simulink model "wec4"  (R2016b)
settings: Solver=ode4  StartTime=0  StopTime=1000  FixedStep=0.005  MaxStep=0.005  RelTol=1e-3  EnableMultiTasking=on
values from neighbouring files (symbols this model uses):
  arAdaptiveLawData = 1/2*zModelSimple.zModelPto.arFreq.*     zModelSimple.zModelPto.arMagnitude./     cos(zModelSimple.zModelPto.arPhase*pi/180+pi/2)    [IMPACT_Control.m]
  arAdaptiveLawDataX = 1/2*zModelSimpleX.zModelPto.arFreq.*         zModelSimpleX.zModelPto.arMagnitude./         cos(zModelSimpleX.zModelPto.arPhase*pi/180+pi/2)    [IMPACT_Control.m]
  arControllerRampGain = [0,0,1,1]    [IMPACT_Control.m]
  arControllerRampTime = [0 rStartRampTime rStartRampTime+rRampTimeLength 8000]    [IMPACT_Control.m]
  arEkfInitialisation = zeros(1,11)    [IMPACT_Control.m]
  arEkfInitialisationX = zeros(1,11)    [IMPACT_Control.m]
  arFrequency = zModelSimple.zModelPto.arFreq    [IMPACT_Control.m]
  arFrequencyRange = zModelSimple.zModelPto.arFreq    [IMPACT_Control.m]
  arFrequencyX = zModelSimpleX.zModelPto.arFreq    [IMPACT_Control.m]
  arImpedance = 1./zModelSimple.zModelPto.arMagnitude./zModelSimple.zModelPto.arFreq    [IMPACT_Control.m]
  arImpedanceX = 1./zModelSimpleX.zModelPto.arMagnitude./zModelSimpleX.zModelPto.arFreq    [IMPACT_Control.m]
  CentralPTOPreload = -1.6113e+07    (= -16113000)    [wecSimInputFile.m]
  F1 = [4.243 2.375 -12.243]    [wecSimInputFile.m]
  F2 = [4.243 -2.375 -12.243]    [wecSimInputFile.m]
  F3 = [-4.243 -2.375 -12.243]    [wecSimInputFile.m]
  F4 = [-4.243 2.375 -12.243]    [wecSimInputFile.m]
  FC = [0 0 -14]    [wecSimInputFile.m]
  iAdaptiveDamping = 0    [wec4IMPACT_Project.m]    (also in IMPACT_Control.m = handles.iAdaptiveDamping; wec1_IMPACT_Project.m; wec2_IMPACT_Project.m; wec3_IMPACT_Project.m)
  iControlType = 2    [wec4IMPACT_Project.m]    (also in IMPACT_Control.m = handles.iControlType; wec1_IMPACT_Project.m = 1; wec2_IMPACT_Project.m = 1; wec3_IMPACT_Project.m = 1)
  iPtoPositionConstraint = 1    [wec4IMPACT_Project.m]    (also in IMPACT_Control.m = handles.iPtoPositionConstraint; wec1_IMPACT_Project.m = 0; wec2_IMPACT_Project.m; wec3_IMPACT_Project.m)
  iSensorNoise = 0    [IMPACT_Control.m]
  m = m+1    (= 2)    [checkParamFile.m]
  PTOrotation = atan((T1(2)-F1(2))/(T1(1)-F1(1)))    [wecSimInputFile.m]
  rCogFloater = -8    [wec4_IMPACT_Model.m]    (also in paramInitial.m = get( handles.edit_rCogFloater, 'String' ); wec1_IMPACT_Model.m = -18; wec2_IMPACT_Model.m = -8.5; wec3_IMPACT_Model.m = -0.7)
  rCogSpar = -36.6    [wec4_IMPACT_Model.m]    (also in paramInitial.m = get( handles.edit_rCogSpar, 'String' ); wec3_IMPACT_Model.m = -21.3; wec3_IMPACT_Model2.m = -21.3)
  rDisplacementLimit = 10.000000    (= 10)    [wec4IMPACT_Project.m]    (also in IMPACT_Control.m = getValue(handles.edit_displacementLimit); wec1_IMPACT_Project.m; wec2_IMPACT_Project.m; wec3_IMPACT_Project.m = 3)
  rDisplacementLimitX = 10.000000    (= 10)    [wec4IMPACT_Project.m]    (also in IMPACT_Control.m = getValue(handles.edit_displacementLimitX); wec1_IMPACT_Project.m = 0; wec2_IMPACT_Project.m; wec3_IMPACT_Project.m = 0)
  rGainForAntiWIndUp = tfControllerDiscrete.rGain    [IMPACT_Control.m]
  rGainForAntiWIndUpX = tfControllerXDiscrete.rGain    [IMPACT_Control.m]
  rMaxForcePto = 300000000.000000    (= 300000000)    [wec4IMPACT_Project.m]    (also in IMPACT_Control.m = getValue(handles.edit_maxForcePto); wec1_IMPACT_Project.m = 1e+15; wec2_IMPACT_Project.m = 1e+15; wec3_IMPACT_Project.m = 1000000000)
  rMinForcePto = -300000000.000000    (= -300000000)    [wec4IMPACT_Project.m]    (also in IMPACT_Control.m = getValue(handles.edit_minForcePto); wec1_IMPACT_Project.m = -1e+15; wec2_IMPACT_Project.m = -1e+15; wec3_IMPACT_Project.m = -1000000000)
  rMooringX = 20000    [wec4_IMPACT_Model.m]    (also in paramInitial.m = get( handles.edit_rMooringX, 'String' ); wec3_IMPACT_Model.m = 10000; wec3_IMPACT_Model2.m = 10000)
  rMooringZ = 10000    [wec4_IMPACT_Model.m]    (also in paramInitial.m = get( handles.edit_rMooringZ, 'String' ); wec3_IMPACT_Model.m = 0; wec3_IMPACT_Model2.m = 0)
  rOutputSampleTime = 0.010000    (= 0.01)    [wec4IMPACT_Project.m]    (also in IMPACT_Control.m = getValue(handles.edit_outputSampleTime); wec1_IMPACT_Project.m; wec2_IMPACT_Project.m; wec3_IMPACT_Project.m)
  rPassiveDampingGain = -604830.000000    (= -604830)    [wec4IMPACT_Project.m]    (also in IMPACT_Control.m = getValue(handles.edit_gainPLD); wec1_IMPACT_Project.m = -214018.1537; wec2_IMPACT_Project.m = -1948070; wec3_IMPACT_Project.m = -519390)
  rPassiveDampingGainX = -278660.000000    (= -278660)    [wec4IMPACT_Project.m]    (also in IMPACT_Control.m = getValue(handles.edit_gainPLDX); wec1_IMPACT_Project.m = 0; wec2_IMPACT_Project.m = 0; wec3_IMPACT_Project.m = 0)
  rTetherPretension = 1.6113e+07    (= 16113000)    [wec4_IMPACT_Model.m]    (also in paramInitial.m = get( handles.edit_rTetherPretension, 'String' ); wec3_IMPACT_Model.m = 0; wec3_IMPACT_Model2.m = 0)
  rTetherSpring = 500000    [wec4_IMPACT_Model.m]    (also in paramInitial.m = get( handles.edit_rTetherSpring, 'String' ); wec3_IMPACT_Model.m = 0; wec3_IMPACT_Model2.m = 0)
  rUpperFrequencyLimit = EKFFloater.upperFreq    [IMPACT_Control.m]
  rXf = 4.243    [wec4AdditionalParams.m]
  rXs = 16.075    [wec4AdditionalParams.m]
  rYf = 2.375    [wec4AdditionalParams.m]
  rYs = 16.075    [wec4AdditionalParams.m]
  rZf = 4.243    [wec4AdditionalParams.m]
  rZs = 2.4350    (= 2.435)    [wec4AdditionalParams.m]
  rZTetherF = 6    [wec4AdditionalParams.m]
  rZTetherS = 2.4350    (= 2.435)    [wec4AdditionalParams.m]
  s = tf('s')    [wec4_IMPACT_Model.m]    (also in IMPACT_Control.m; wec1_IMPACT_Model.m; wec2_IMPACT_Model.m; wec3_IMPACT_Model.m)
  SidePTO1Preload = PreloadPTOCorner    (= 0)    [wecSimInputFile.m]
  SidePTO2Preload = PreloadPTOCorner    (= 0)    [wecSimInputFile.m]
  SidePTO3Preload = PreloadPTOCorner    (= 0)    [wecSimInputFile.m]
  SidePTO4Preload = PreloadPTOCorner    (= 0)    [wecSimInputFile.m]
  simu = simulationClass()    [wecSimInputFile.m]
  T1 = [16.075 16.075 -34.165]    [wecSimInputFile.m]
  T2 = [16.075 -16.075 -34.165]    [wecSimInputFile.m]
  T3 = [-16.075 -16.075 -34.165]    [wecSimInputFile.m]
  T4 = [-16.075 16.075 -34.165]    [wecSimInputFile.m]
  TC = [0 0 -34.165]    [wecSimInputFile.m]
  waves = waveClass('irregular')    [wecSimInputFile.m]
  Z = magPhaseToComplex(zModelTf)    [IMPACT_Control.m]
undefined symbols (not defined in the file or in its folder): arControllerDiscreteDen, arControllerDiscreteNum, arControllerDiscreteXDen, arControllerDiscreteXNum, arExcForceFloaterDen, arExcForceFloaterNum, arExcForceFloaterXDen, arExcForceFloaterXNum, arExcForceSparDen, arExcForceSparNum, arExcForceSparXDen, arExcForceSparXNum, arFexcFloaterDen, arFexcFloaterNum, arFexcFloaterXDen, arFexcFloaterXNum, arFexcSparDen, arFexcSparNum, arFexcSparXDen, arFexcSparXNum, Body, body, constraint, CTTime, deg, Elements, geometry, IRKB, kg, lenJ, mooring, N, pto, rAccelerationGainFloater, rAccelerationGainFloaterX, rAccelerationGainSpar, rAccelerationGainSparX, rad, rBuoyancyGainFloater, rBuoyancyGainFloaterX, rBuoyancyGainSpar, rBuoyancyGainSparX, rDampingGainFloater, rDampingGainFloaterX, rDampingGainSpar, rDampingGainSparX, Rigid, rMaxFocePto, wec4_float, wec4_reactor, WECSim_Lib, X, Y
libraries: nesl_utility x380, sm_lib x170, vrlib x91, simulink x12, WECSim_Lib x4
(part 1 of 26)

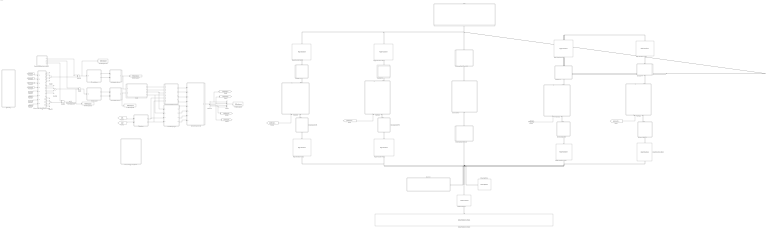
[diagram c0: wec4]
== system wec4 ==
  Central tether : Subsystem
  Demux1 : Demux
  EKFs : Subsystem
  Excitation force : Subsystem
  Excitation force1 : Subsystem
  Float : Subsystem  AncestorBlock=WECSim_Lib/Body Elements/Rigid Body  Variant=on
  Floating (3DOF) : WECSim_Lib/Constraints/Floating (3DOF)  constraint=constraint(1)
  Force of Tether in x,y and z1 : Subsystem
  Force of the four PTOs in x,y and z : Subsystem
  Gimbal F1 : Subsystem  AncestorBlock=WECSim_Lib/Constraints/Rotational
  Gimbal F2 : Subsystem  AncestorBlock=WECSim_Lib/Constraints/Rotational
  Gimbal F3 : Subsystem  AncestorBlock=WECSim_Lib/Constraints/Rotational
  Gimbal F4 : Subsystem  AncestorBlock=WECSim_Lib/Constraints/Rotational
  Global Reference Frame : WECSim_Lib/Frames/Global Reference Frame  waves=waves  simu=simu
  MooringMatrix : WECSim_Lib/Moorings/MooringMatrix  mooring=mooring(1)
  Mux5 : Mux
  OVT : Subsystem
  PTO P1F1 : Subsystem
  PTO P2F2 : Subsystem
  PTO P3F3 : Subsystem
  PTO P4F4 : Subsystem
  Reactor : Subsystem  AncestorBlock=WECSim_Lib/Body Elements/Rigid Body  Variant=on
  Rigid Transform F1P1 : sm_lib/Frames and Transforms/Rigid Transform  TranslationMethod=None  TranslationStandardOffset=0  TranslationLengthUnit=m  TranslationStandardAxis=+Z  TranslationCartesianOffset=[0 0 0]  TranslationROffset=0  TranslationROffsetUnits=m  TranslationZOffset=0  TranslationZOffsetUnits=m  TranslationThetaOffset=0  TranslationThetaOffsetUnits=deg  RotationMethod=StandardAxis  RotationAngleUnits=rad  RotationStandardAxis=+Z  RotationAngle=PTOrotation  RotationArbitraryAxis=[0 0 1]  FollAlignAxisA=+X  BaseAlignAxisA=+Y  FollAlignAxisB=+Y  BaseAlignAxisB=+Z  RotationSequenceAxes=FollowerAxes  RotationSequence=XYX  RotationSequenceAngles=[0 0 0]  RotationSequenceAnglesUnits=deg  RotationMatrix=[1 0 0; 0 1 0; 0 0 1]
  Rigid Transform F2P2 : sm_lib/Frames and Transforms/Rigid Transform  TranslationMethod=None  TranslationStandardOffset=0  TranslationLengthUnit=m  TranslationStandardAxis=+Z  TranslationCartesianOffset=[0 0 0]  TranslationROffset=0  TranslationROffsetUnits=m  TranslationZOffset=0  TranslationZOffsetUnits=m  TranslationThetaOffset=0  TranslationThetaOffsetUnits=deg  RotationMethod=StandardAxis  RotationAngleUnits=rad  RotationStandardAxis=+Z  RotationAngle=-PTOrotation  RotationArbitraryAxis=[0 0 1]  FollAlignAxisA=+X  BaseAlignAxisA=+Y  FollAlignAxisB=+Y  BaseAlignAxisB=+Z  RotationSequenceAxes=FollowerAxes  RotationSequence=XYX  RotationSequenceAngles=[0 0 0]  RotationSequenceAnglesUnits=deg  RotationMatrix=[1 0 0; 0 1 0; 0 0 1]
  Rigid Transform F3P3 : sm_lib/Frames and Transforms/Rigid Transform  TranslationMethod=None  TranslationStandardOffset=0  TranslationLengthUnit=m  TranslationStandardAxis=+Z  TranslationCartesianOffset=[0 0 0]  TranslationROffset=0  TranslationROffsetUnits=m  TranslationZOffset=0  TranslationZOffsetUnits=m  TranslationThetaOffset=0  TranslationThetaOffsetUnits=deg  RotationMethod=StandardAxis  RotationAngleUnits=rad  RotationStandardAxis=+Z  RotationAngle=-pi+PTOrotation  RotationArbitraryAxis=[0 0 1]  FollAlignAxisA=+X  BaseAlignAxisA=+Y  FollAlignAxisB=+Y  BaseAlignAxisB=+Z  RotationSequenceAxes=FollowerAxes  RotationSequence=XYX  RotationSequenceAngles=[0 0 0]  RotationSequenceAnglesUnits=deg  RotationMatrix=[1 0 0; 0 1 0; 0 0 1]
  Rigid Transform F4P4 : sm_lib/Frames and Transforms/Rigid Transform  TranslationMethod=None  TranslationStandardOffset=0  TranslationLengthUnit=m  TranslationStandardAxis=+Z  TranslationCartesianOffset=[0 0 0]  TranslationROffset=0  TranslationROffsetUnits=m  TranslationZOffset=0  TranslationZOffsetUnits=m  TranslationThetaOffset=0  TranslationThetaOffsetUnits=deg  RotationMethod=StandardAxis  RotationAngleUnits=rad  RotationStandardAxis=+Z  RotationAngle=pi-PTOrotation  RotationArbitraryAxis=[0 0 1]  FollAlignAxisA=+X  BaseAlignAxisA=+Y  FollAlignAxisB=+Y  BaseAlignAxisB=+Z  RotationSequenceAxes=FollowerAxes  RotationSequence=XYX  RotationSequenceAngles=[0 0 0]  RotationSequenceAnglesUnits=deg  RotationMatrix=[1 0 0; 0 1 0; 0 0 1]
  Rigid Transform P1F1 : sm_lib/Frames and Transforms/Rigid Transform  TranslationMethod=None  TranslationStandardOffset=0  TranslationLengthUnit=m  TranslationStandardAxis=+Z  TranslationCartesianOffset=[0 0 0]  TranslationROffset=0  TranslationROffsetUnits=m  TranslationZOffset=0  TranslationZOffsetUnits=m  TranslationThetaOffset=0  TranslationThetaOffsetUnits=deg  RotationMethod=StandardAxis  RotationAngleUnits=rad  RotationStandardAxis=+Z  RotationAngle=PTOrotation  RotationArbitraryAxis=[0 0 1]  FollAlignAxisA=+X  BaseAlignAxisA=+Y  FollAlignAxisB=+Y  BaseAlignAxisB=+Z  RotationSequenceAxes=FollowerAxes  RotationSequence=XYX  RotationSequenceAngles=[0 0 0]  RotationSequenceAnglesUnits=deg  RotationMatrix=[1 0 0; 0 1 0; 0 0 1]
  Rigid Transform P2F2 : sm_lib/Frames and Transforms/Rigid Transform  TranslationMethod=None  TranslationStandardOffset=0  TranslationLengthUnit=m  TranslationStandardAxis=+Z  TranslationCartesianOffset=[0 0 0]  TranslationROffset=0  TranslationROffsetUnits=m  TranslationZOffset=0  TranslationZOffsetUnits=m  TranslationThetaOffset=0  TranslationThetaOffsetUnits=deg  RotationMethod=StandardAxis  RotationAngleUnits=rad  RotationStandardAxis=+Z  RotationAngle=-PTOrotation  RotationArbitraryAxis=[0 0 1]  FollAlignAxisA=+X  BaseAlignAxisA=+Y  FollAlignAxisB=+Y  BaseAlignAxisB=+Z  RotationSequenceAxes=FollowerAxes  RotationSequence=XYX  RotationSequenceAngles=[0 0 0]  RotationSequenceAnglesUnits=deg  RotationMatrix=[1 0 0; 0 1 0; 0 0 1]
  Rigid Transform P3F3 : sm_lib/Frames and Transforms/Rigid Transform  TranslationMethod=None  TranslationStandardOffset=0  TranslationLengthUnit=m  TranslationStandardAxis=+Z  TranslationCartesianOffset=[0 0 0]  TranslationROffset=0  TranslationROffsetUnits=m  TranslationZOffset=0  TranslationZOffsetUnits=m  TranslationThetaOffset=0  TranslationThetaOffsetUnits=deg  RotationMethod=StandardAxis  RotationAngleUnits=rad  RotationStandardAxis=+Z  RotationAngle=-pi+PTOrotation  RotationArbitraryAxis=[0 0 1]  FollAlignAxisA=+X  BaseAlignAxisA=+Y  FollAlignAxisB=+Y  BaseAlignAxisB=+Z  RotationSequenceAxes=FollowerAxes  RotationSequence=XYX  RotationSequenceAngles=[0 0 0]  RotationSequenceAnglesUnits=deg  RotationMatrix=[1 0 0; 0 1 0; 0 0 1]
  Rigid Transform P4F4 : sm_lib/Frames and Transforms/Rigid Transform  TranslationMethod=None  TranslationStandardOffset=0  TranslationLengthUnit=m  TranslationStandardAxis=+Z  TranslationCartesianOffset=[0 0 0]  TranslationROffset=0  TranslationROffsetUnits=m  TranslationZOffset=0  TranslationZOffsetUnits=m  TranslationThetaOffset=0  TranslationThetaOffsetUnits=deg  RotationMethod=StandardAxis  RotationAngleUnits=rad  RotationStandardAxis=+Z  RotationAngle=pi-PTOrotation  RotationArbitraryAxis=[0 0 1]  FollAlignAxisA=+X  BaseAlignAxisA=+Y  FollAlignAxisB=+Y  BaseAlignAxisB=+Z  RotationSequenceAxes=FollowerAxes  RotationSequence=XYX  RotationSequenceAngles=[0 0 0]  RotationSequenceAnglesUnits=deg  RotationMatrix=[1 0 0; 0 1 0; 0 0 1]
  Subsystem : Subsystem
  Sum10 : Sum
  Sum12 : Sum  Inputs=+--+
  Sum13 : Sum
  Sum16 : Sum  Inputs=--++
  Sum2 : Sum
  Sum9 : Sum  Inputs=++++
  Terminator3 Rise of the machines : Terminator
  To Workspace10 : ToWorkspace  VariableName=arForceVerticalFloater  SampleTime=rOutputSampleTime
  To Workspace21 : ToWorkspace  VariableName=arTotalPtoForceX  SampleTime=rOutputSampleTime
  To Workspace5 : ToWorkspace  VariableName=arPtoForceDemand  SampleTime=rOutputSampleTime
  To Workspace7 : ToWorkspace  VariableName=arCombinedForceZ  SampleTime=rOutputSampleTime
  To Workspace8 : ToWorkspace  VariableName=arCominedForceX  SampleTime=rOutputSampleTime
  Universal Joint Central : Subsystem  AncestorBlock=WECSim_Lib/Constraints/Rotational
  Universal Joint Central1 : Subsystem  AncestorBlock=WECSim_Lib/Constraints/Rotational
  Universal Joint P1 : Subsystem  AncestorBlock=WECSim_Lib/Constraints/Rotational
  Universal Joint P2 : Subsystem  AncestorBlock=WECSim_Lib/Constraints/Rotational
  Universal Joint P3 : Subsystem  AncestorBlock=WECSim_Lib/Constraints/Rotational
  Universal Joint P4 : Subsystem  AncestorBlock=WECSim_Lib/Constraints/Rotational
  X Excitation : Subsystem
  Z excitation : Subsystem
  controllerSwitching : Subsystem
  "force, energy, and power" : Subsystem
  geometry : Subsystem
  linearDamping1 : Subsystem
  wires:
  [ptoForceDemand1] -> PTO P1F1/1(P1F1_force)
  [ptoForceDemand2] -> PTO P2F2/1(P2F2_force)
  [ptoForceDemand3] -> PTO P3F3/1(P3F3_force)
  [ptoForceDemand4] -> PTO P4F4/1(P4F4_force)
  Force of the four PTOs in x,y and z/7(Fx3) -> Sum16/3
  Force of the four PTOs in x,y and z/8(Fx4) -> Sum16/4
  Force of the four PTOs in x,y and z/6(Fx2) -> Sum16/2
  Force of the four PTOs in x,y and z/1(Fz1) -> Sum9/1
  Force of the four PTOs in x,y and z/3(Fz3) -> Sum9/3
  Force of the four PTOs in x,y and z/4(Fz4) -> Sum9/4
  Force of the four PTOs in x,y and z/2(Fz2) -> Sum9/2
  Force of the four PTOs in x,y and z/10(Fy2) -> Sum12/2
  Force of the four PTOs in x,y and z/12(Fy4) -> Sum12/4
  Force of the four PTOs in x,y and z/9(Fy1) -> Sum12/1
  Force of the four PTOs in x,y and z/11(Fy3) -> Sum12/3
  Sum9/1 -> Sum10/2
  Force of the four PTOs in x,y and z/5(Fx1) -> Sum16/1
  Sum12/1 -> Sum13/2
  Force of Tether in x,y and z1/2(FRx) -> Sum2/1
  Force of Tether in x,y and z1/3(FRy) -> Sum13/1
  Force of Tether in x,y and z1/1(FRz) -> Sum10/1
  Sum10/1 -> Z excitation/1(PTO force Z), To Workspace10/1
  Sum16/1 -> To Workspace21/1, Sum2/2
  Sum2/1 -> X Excitation/1(PTO force X)
  Sum13/1 -> Terminator3 Rise of the machines/1
  EKFs/2(referenceVelocityZ) -> OVT/2(vref_z)
  Mux5/1 -> To Workspace5/1
  EKFs/3(ekfFreqZ) -> linearDamping1/1(ekfFrequencyZ), OVT/3(ekfFreqZ)
  EKFs/1(referenceVelocityX) -> OVT/1(vref_x)
  Demux1/4 -> [ptoForceDemand4], Mux5/4
  Demux1/3 -> [ptoForceDemand3], Mux5/3
  Demux1/2 -> [ptoForceDemand2], Mux5/2
  Demux1/1 -> [ptoForceDemand1], Mux5/1
  Excitation force/1(Combined Fexc) -> EKFs/1(excitationForceZ), To Workspace7/1
  Z excitation/1(floaterExcitation) -> Excitation force/1(Fexc floater)
  Z excitation/2(SparExcitation) -> Excitation force/2(Fexc spar)
  Excitation force1/1(Combined Fexc X) -> To Workspace8/1, EKFs/2(excitationForceX)
  X Excitation/1(floaterExcitation) -> Excitation force1/1(Fexc floater)
  X Excitation/2(SparExcitation) -> Excitation force1/2(Fexc spar)
  [gamma1] -> Force of the four PTOs in x,y and z/1(gamma1)
  [gamma3] -> Force of the four PTOs in x,y and z/3(gamma3)
  [kappa1] -> Force of the four PTOs in x,y and z/5(alpha1)
  [kappa3] -> Force of the four PTOs in x,y and z/7(alpha3)
  [gamma4] -> Force of the four PTOs in x,y and z/4(gamma4)
  [gamma2] -> Force of the four PTOs in x,y and z/2(gamma2)
  [kappa2] -> Force of the four PTOs in x,y and z/6(alpha2)
  [kappa4] -> Force of the four PTOs in x,y and z/8(alpha4)
  controllerSwitching/1(forceDemand) -> Demux1/1
  EKFs/4(ekfFreqX) -> linearDamping1/2(ekfFrequencyX), OVT/4(ekfFreqX)
  OVT/4(forceDemand4) -> controllerSwitching/4(ovtForceDemand4)
  OVT/3(forceDemand3) -> controllerSwitching/3(ovtForceDemand3)
  OVT/2(forceDemand2) -> controllerSwitching/2(ovtForceDemand2)
  OVT/1(forceDemand1) -> controllerSwitching/1(ovtForceDemand1)
  linearDamping1/1(forceDemand1) -> controllerSwitching/5(linearDampingForce1)
  linearDamping1/2(forceDemand2) -> controllerSwitching/6(linearDampingForce2)
  linearDamping1/3(forceDemand3) -> controllerSwitching/7(linearDampingForce3)
  linearDamping1/4(forceDemand4) -> controllerSwitching/8(linearDampingForce4)
  [vel1] -> Subsystem/1(Vel floater 6x1)
  [vel2] -> Subsystem/2(Vel Spar 6x1)
  Subsystem/1("Rel. vel. X ") -> OVT/5(Rel. vel X), linearDamping1/3(Rel. vel X)
  Subsystem/2(Rel. vel. Z) -> OVT/6(Rel. vel. Z), linearDamping1/4(Rel. vel. Z)
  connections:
  Rigid Transform P2F2/LConn1 -- Rigid Transform P1F1/LConn1 -- Rigid Transform P4F4/LConn1 -- Rigid Transform P3F3/LConn1 -- Floating (3DOF)/RConn1 -- Reactor/RConn1 -- MooringMatrix/LConn1 -- Universal Joint Central/LConn1
  Float/RConn1 -- Universal Joint Central1/RConn1 -- Rigid Transform F4P4/LConn1 -- Rigid Transform F3P3/LConn1 -- Rigid Transform F2P2/LConn1 -- Rigid Transform F1P1/LConn1
  PTO P3F3/LConn1 -- Universal Joint P3/RConn1
  Universal Joint P1/LConn1 -- Rigid Transform P1F1/RConn1
  Rigid Transform F1P1/RConn1 -- Gimbal F1/RConn1
  Gimbal F1/LConn1 -- PTO P1F1/RConn1
  PTO P1F1/LConn1 -- Universal Joint P1/RConn1
  Rigid Transform F2P2/RConn1 -- Gimbal F2/RConn1
  Universal Joint P2/LConn1 -- Rigid Transform P2F2/RConn1
  Rigid Transform F3P3/RConn1 -- Gimbal F3/RConn1
  Rigid Transform F4P4/RConn1 -- Gimbal F4/RConn1
  Universal Joint P4/LConn1 -- Rigid Transform P4F4/RConn1
  Gimbal F2/LConn1 -- PTO P2F2/RConn1
  PTO P2F2/LConn1 -- Universal Joint P2/RConn1
  Universal Joint Central1/LConn1 -- Central tether/RConn1
  Central tether/LConn1 -- Universal Joint Central/RConn1
  Gimbal F3/LConn1 -- PTO P3F3/RConn1
  Gimbal F4/LConn1 -- PTO P4F4/RConn1
  Rigid Transform P3F3/RConn1 -- Universal Joint P3/LConn1
  PTO P4F4/LConn1 -- Universal Joint P4/RConn1
  Global Reference Frame/RConn1 -- Floating (3DOF)/LConn1

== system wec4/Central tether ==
  CentralTether_preload : Constant  Value=CentralPTOPreload
  PTO Central visu : Subsystem  AncestorBlock=WECSim_Lib/Body Elements/Rigid Body  Variant=on
  Terminator PTO Central : Terminator
  Translational PTO Actuation Force Central : WECSim_Lib/PTOs/Translational PTO Actuation Force  pto=pto(5)
  Conn1 : PMIOPort  Port=1  Side=Right
  Conn2 : PMIOPort  Port=2  Side=Left
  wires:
  CentralTether_preload/1 -> Translational PTO Actuation Force Central/1
  Translational PTO Actuation Force Central/1 -> Terminator PTO Central/1
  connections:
  Translational PTO Actuation Force Central/RConn1 -- PTO Central visu/RConn1 -- Conn1/RConn1
  Translational PTO Actuation Force Central/LConn1 -- Conn2/RConn1

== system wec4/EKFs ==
  excitationForceZ : Inport
  excitationForceX : Inport  Port=2
  Abs1 : Abs
  Abs2 : Abs
  Clock1 : Clock
  Clock3 : Clock
  Constant1 : Constant  Value=arEkfInitialisation
  Constant2 : Constant  Value=arEkfInitialisationX
  Divide1 : Product  Inputs=**
  Divide4 : Product  Inputs=**
  EKF : MATLAB Function  TreatAsAtomicUnit=on
  EKF1 : MATLAB Function  TreatAsAtomicUnit=on
  Ramp gain : Lookup_n-D  NumberOfTableDimensions=1  BreakpointsForDimension1=[0 5 10 8000]  Table=[0 0 1 1]  InternalRulePriority=Speed  RndMeth=Simplest
  Ramp gain1 : Lookup_n-D  NumberOfTableDimensions=1  BreakpointsForDimension1=[0 5 10 8000]  Table=[0 0 1 1]  InternalRulePriority=Speed  RndMeth=Simplest
  Rate Transition1 : RateTransition  OutPortSampleTimeMultiple=0.01  OutPortSampleTime=rControllerSampleTime
  Rate Transition2 : RateTransition  OutPortSampleTimeMultiple=0.01  OutPortSampleTime=rControllerSampleTime
  Saturation1 : Saturate  UpperLimit=rUpperFrequencyLimit  LowerLimit=0  LinearizeAsGain=off
  Saturation2 : Saturate  UpperLimit=rUpperFrequencyLimit  LowerLimit=0  LinearizeAsGain=off
  Terminator3 : Terminator
  Terminator4 : Terminator
  To Workspace1 : ToWorkspace  VariableName=arPhi0Z  SampleTime=rOutputSampleTime
  To Workspace4 : ToWorkspace  VariableName=arEstimatedExcitationForceZ  SampleTime=rOutputSampleTime
  To Workspace5 : ToWorkspace  VariableName=arEkfAmplitudeZ  SampleTime=rOutputSampleTime
  To Workspace6 : ToWorkspace  VariableName=arEkfFrequencyZ  SampleTime=rOutputSampleTime
  To Workspace7 : ToWorkspace  VariableName=arEstimatedExcitationForceX  SampleTime=rOutputSampleTime
  To Workspace8 : ToWorkspace  VariableName=arEkfAmplitudeX  SampleTime=rOutputSampleTime
  To Workspace9 : ToWorkspace  VariableName=arEkfFrequencyX  SampleTime=rOutputSampleTime
  Transfer Fcn{1..2,4..7,9..10} (8 alike) : TransferFcn  Numerator=[400]  Denominator=[1 40 400]
  V ref X : Subsystem
  "V ref Z " : Subsystem
  referenceVelocityX : Outport
  referenceVelocityZ : Outport  Port=2
  ekfFreqZ : Outport  Port=3
  ekfFreqX : Outport  Port=4
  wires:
  Clock1/1 -> Ramp gain1/1
  Ramp gain1/1 -> Divide1/1
  excitationForceX/1 -> Divide1/2
  Clock3/1 -> Ramp gain/1
  Transfer Fcn5/1 -> To Workspace5/1, "V ref Z "/3(ekfAmplitude)
  EKF/3(rFrequencyOutput) -> Transfer Fcn2/1
  Saturation1/1 -> "V ref Z "/2(ekfFrequency), ekfFreqZ/1, To Workspace6/1
  Constant1/1 -> EKF/2(arEkfInitialisation)
  "V ref Z "/1(referenceVelocity) -> referenceVelocityZ/1
  Abs1/1 -> Saturation1/1
  Transfer Fcn2/1 -> Abs1/1
  excitationForceZ/1 -> Divide4/2
  EKF/1(rPhi0Output) -> To Workspace1/1, Transfer Fcn4/1
  Divide4/1 -> Rate Transition1/1, To Workspace4/1
  Ramp gain/1 -> Divide4/1
  EKF/2(rPhi0StarOutput) -> Transfer Fcn1/1
  Transfer Fcn4/1 -> "V ref Z "/1(phiOut)
  Rate Transition1/1 -> EKF/1(rEstimatedExcitationForce)
  V ref X/1(referenceVelocity) -> referenceVelocityX/1
  EKF/4(rAmplitudeOutput) -> Transfer Fcn5/1
  EKF1/3(rFrequencyOutput) -> Transfer Fcn7/1
  Transfer Fcn10/1 -> V ref X/3(ekfAmplitude), To Workspace8/1
  Transfer Fcn9/1 -> V ref X/1(phiOut)
  Abs2/1 -> Saturation2/1
  Constant2/1 -> EKF1/2(arEkfInitialisation)
  Transfer Fcn6/1 -> Terminator4/1
  EKF1/4(rAmplitudeOutput) -> Transfer Fcn10/1
  EKF1/1(rPhi0Output) -> Transfer Fcn9/1
  Transfer Fcn7/1 -> Abs2/1
  Divide1/1 -> Rate Transition2/1, To Workspace7/1
  EKF1/2(rPhi0StarOutput) -> Transfer Fcn6/1
  Rate Transition2/1 -> EKF1/1(rEstimatedExcitationForce)
  Transfer Fcn1/1 -> Terminator3/1
  Saturation2/1 -> To Workspace9/1, ekfFreqX/1, V ref X/2(ekfFrequency)

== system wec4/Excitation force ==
  Fexc floater : Inport
  Fexc spar : Inport  Port=2
  Add : Sum
  Clock3 : Clock
  Divide1 : Product  Inputs=**
  Divide4 : Product  Inputs=**
  Fexc Floater : TransferFcn  Numerator=arFexcFloaterNum  Denominator=arFexcFloaterDen
  Fexc Spar : TransferFcn  Numerator=arFexcSparNum  Denominator=arFexcSparDen
  Ramp gain : Lookup_n-D  NumberOfTableDimensions=1  BreakpointsForDimension1=[0 5 10 8000]  Table=[0 0 1 1]  InternalRulePriority=Speed  RndMeth=Simplest
  Ramp gain1 : Lookup_n-D  NumberOfTableDimensions=1  BreakpointsForDimension1=[0 20 25 8000]  Table=[0 0 1 1]  InternalRulePriority=Speed  RndMeth=Simplest
  Combined Fexc : Outport
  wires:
  Fexc floater/1 -> Divide4/2
  Fexc Floater/1 -> Add/1
  Fexc Spar/1 -> Add/2
  Add/1 -> Combined Fexc/1
  Clock3/1 -> Ramp gain1/1, Ramp gain/1
  Ramp gain/1 -> Divide4/1
  Divide4/1 -> Fexc Floater/1
  Ramp gain1/1 -> Divide1/2
  Divide1/1 -> Fexc Spar/1
  Fexc spar/1 -> Divide1/1

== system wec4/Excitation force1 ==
  Fexc floater : Inport
  Fexc spar : Inport  Port=2
  Add : Sum
  Clock3 : Clock
  Divide1 : Product  Inputs=**
  Divide4 : Product  Inputs=**
  Fexc Floater X : TransferFcn  Numerator=arFexcFloaterXNum  Denominator=arFexcFloaterXDen
  Fexc Spar X : TransferFcn  Numerator=arFexcSparXNum  Denominator=arFexcSparXDen
  Ramp gain : Lookup_n-D  NumberOfTableDimensions=1  BreakpointsForDimension1=[0 5 10 8000]  Table=[0 0 1 1]  InternalRulePriority=Speed  RndMeth=Simplest
  Ramp gain1 : Lookup_n-D  NumberOfTableDimensions=1  BreakpointsForDimension1=[0 20 25 8000]  Table=[0 0 1 1]  InternalRulePriority=Speed  RndMeth=Simplest
  Combined Fexc X : Outport
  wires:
  Divide1/1 -> Fexc Spar X/1
  Ramp gain1/1 -> Divide1/2
  Divide4/1 -> Fexc Floater X/1
  Ramp gain/1 -> Divide4/1
  Clock3/1 -> Ramp gain1/1, Ramp gain/1
  Add/1 -> Combined Fexc X/1
  Fexc Spar X/1 -> Add/2
  Fexc Floater X/1 -> Add/1
  Fexc floater/1 -> Divide4/2
  Fexc spar/1 -> Divide1/1

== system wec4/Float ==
  note: 1) Add Subsystem or Model blocks as valid variant choices. 2) You cannot connect blocks at this level. At simulation, connectivity is automatically determined, based on the active variant and port name matching.
  Hydrodynamic Body : Subsystem  VariantControl=sv_b1_hydroBody
  Non-Hydro Body : Subsystem  VariantControl=sv_b1_nonHydroBody
  Conn : PMIOPort  Port=1  Side=Right

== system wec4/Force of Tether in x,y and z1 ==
  Constant3 : Constant  Value=-rTetherPretension
  Dzs/2 (2) : Constant  Value=TC(3)
  Dzs/2 (2)1 : Constant  Value=FC(3)
  Gain : Gain  Gain=-rTetherSpring
  Gain1 : Gain  Gain=180/pi
  Math Function{,1..5} (6 alike) : Math  Operator=square
  Mux1 : Mux  Inputs=2
  Mux3 : Mux  Inputs=2
  Mux4 : Mux  Inputs=2
  Product{,1..3} (4 alike) : Product
  Scope{1..4,6,11..12} (7 alike) : Scope
  Selector11 : Selector  InputPortWidth=6  IndexOptions=Index vector (dialog)  Indices=1  OutputSizes=1
  Selector12 : Selector  InputPortWidth=6  IndexOptions=Index vector (dialog)  Indices=2  OutputSizes=1
  Selector13 : Selector  InputPortWidth=6  IndexOptions=Index vector (dialog)  Indices=3  OutputSizes=1
  Selector14 : Selector  InputPortWidth=6  IndexOptions=Index vector (dialog)  Indices=1  OutputSizes=1
  Selector15 : Selector  InputPortWidth=6  IndexOptions=Index vector (dialog)  Indices=2  OutputSizes=1
  Selector16 : Selector  InputPortWidth=6  IndexOptions=Index vector (dialog)  Indices=3  OutputSizes=1
  Sqrt : Sqrt
  Sqrt1 : Sqrt
  Subsystem2 : Subsystem
  Sum10 : Sum
  Sum11 : Sum  Inputs=-+
  Sum2 : Sum  Inputs=-+
  Sum31 : Sum  Inputs=+++
  Sum{4,6..8} (4 alike) : Sum  Inputs=+-
  Sum9 : Sum  Inputs=+++
  Trigonometric Function : Trigonometry  Operator=atan2
  Trigonometric Function1 : Trigonometry  Operator=atan2
  Trigonometric Function2 : Trigonometry  Operator=cos
  Trigonometric Function3 : Trigonometry  Operator=cos
  Trigonometric Function4 : Trigonometry
  Trigonometric Function5 : Trigonometry
  FRz : Outport
  FRx : Outport  Port=2
  FRy : Outport  Port=3
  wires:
  Trigonometric Function1/1 -> Trigonometric Function5/1, Mux1/2, Trigonometric Function3/1
  Trigonometric Function/1 -> Mux1/1, Trigonometric Function4/1, Trigonometric Function2/1
  Trigonometric Function2/1 -> Product/1
  Trigonometric Function3/1 -> Product/2
  Product/1 -> Product2/2  "Proportion of force in Z direction"
  Trigonometric Function4/1 -> Product1/2
  Math Function/1 -> Sum31/1
  Math Function2/1 -> Sum31/2
  Math Function1/1 -> Sum31/3
  Sum31/1 -> Sqrt/1
  Sqrt/1 -> Mux3/2, Scope4/1, Mux4/2, Sum2/2
  Product1/1 -> FRx/1
  Product3/1 -> FRy/1
  Trigonometric Function5/1 -> Product3/2
  Subsystem2/1(x_total) -> Math Function/1, Trigonometric Function/1
  Mux1/1 -> Gain1/1
  Gain1/1 -> Scope1/1
  Subsystem2/2(y_total) -> Math Function2/1, Trigonometric Function1/1
  Subsystem2/3(z_total) -> Math Function1/1, Trigonometric Function/2, Trigonometric Function1/2
  Sum2/1 -> Scope2/1, Gain/1  "new length minus original length"
  Sum4/1 -> Scope3/1, Mux3/1, Sum2/1
  Dzs/2 (2)1/1 -> Sum4/1
  Dzs/2 (2)/1 -> Sum4/2
  Mux3/1 -> Scope6/1
  [disp2] -> Selector16/1, Selector15/1, Selector14/1
  [disp1] -> Selector13/1, Selector12/1, Selector11/1
  Sum8/1 -> Math Function4/1
  Sum7/1 -> Math Function5/1
  Sum6/1 -> Math Function3/1
  Selector14/1 -> Sum6/2
  Selector11/1 -> Sum6/1
  Selector12/1 -> Sum7/1
  Selector15/1 -> Sum7/2
  Selector13/1 -> Sum8/1
  Selector16/1 -> Sum8/2
  Sqrt1/1 -> Mux4/1
  Sum9/1 -> Sqrt1/1
  Math Function5/1 -> Sum9/2
  Math Function3/1 -> Sum9/1
  Math Function4/1 -> Sum9/3
  Mux4/1 -> Scope11/1
  Gain/1 -> Sum10/1
  Sum11/1 -> Scope12/1, FRz/1
  Product2/1 -> Sum11/2
  Constant3/1 -> Sum11/1, Sum10/2  "Pre-load"
  Sum10/1 -> Product2/1, Product1/1, Product3/1  "Force of tether"

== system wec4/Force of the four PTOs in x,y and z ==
  gamma1 : Inport
  gamma2 : Inport  Port=2
  gamma3 : Inport  Port=3
  gamma4 : Inport  Port=4
  alpha1 : Inport  Port=5
  alpha2 : Inport  Port=6
  alpha3 : Inport  Port=7
  alpha4 : Inport  Port=8
  Product{1..16} (16 alike) : Product
  To Workspace22 : ToWorkspace  VariableName=Fx1  SampleTime=rOutputSampleTime
  Trigonometric Function{,1..3,7..8,11,15} (8 alike) : Trigonometry
  Trigonometric Function{4..6,9..10,12..14} (8 alike) : Trigonometry  Operator=cos
  Fz1 : Outport
  Fz2 : Outport  Port=2
  Fz3 : Outport  Port=3
  Fz4 : Outport  Port=4
  Fx1 : Outport  Port=5
  Fx2 : Outport  Port=6
  Fx3 : Outport  Port=7
  Fx4 : Outport  Port=8
  Fy1 : Outport  Port=9
  Fy2 : Outport  Port=10
  Fy3 : Outport  Port=11
  Fy4 : Outport  Port=12
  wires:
  gamma3/1 -> Trigonometric Function6/1, Trigonometric Function3/1
  Product5/1 -> Fz3/1
  [ptoForce3] -> Product5/1
  [ptoForce2] -> Product6/1
  [ptoForce4] -> Product4/1
  Product6/1 -> Fz2/1
  Product7/1 -> Fz1/1
  [ptoForce1] -> Product7/1
  gamma2/1 -> Trigonometric Function14/1, Trigonometric Function2/1
  Trigonometric Function/1 -> Product7/2
  Trigonometric Function1/1 -> Product4/2
  Trigonometric Function3/1 -> Product5/2
  Product4/1 -> Fz4/1
  Trigonometric Function2/1 -> Product6/2
  [ptoForce1] -> Product8/1
  gamma1/1 -> Trigonometric Function4/1, Trigonometric Function/1
  Trigonometric Function4/1 -> Product8/2
  Product12/1 -> Fy1/1
  Trigonometric Function8/1 -> Product12/1
  Product8/1 -> Product12/2, Product13/2
  Product13/1 -> Fx1/1, To Workspace22/1
  alpha1/1 -> Trigonometric Function8/1, Trigonometric Function12/1
  Trigonometric Function12/1 -> Product13/1
  [ptoForce3] -> Product3/1
  Trigonometric Function6/1 -> Product3/2
  Product1/1 -> Fy3/1
  Trigonometric Function7/1 -> Product1/1
  Product3/1 -> Product2/2, Product1/2
  Product2/1 -> Fx3/1
  alpha3/1 -> Trigonometric Function5/1, Trigonometric Function7/1
  Trigonometric Function5/1 -> Product2/1
  gamma4/1 -> Trigonometric Function10/1, Trigonometric Function1/1
  Trigonometric Function10/1 -> Product11/2
  Trigonometric Function11/1 -> Product9/1
  Product11/1 -> Product9/2, Product10/2
  Product10/1 -> Fx4/1
  alpha4/1 -> Trigonometric Function11/1, Trigonometric Function9/1
  Trigonometric Function9/1 -> Product10/1
  Product9/1 -> Fy4/1
  [ptoForce2] -> Product16/1
  Trigonometric Function14/1 -> Product16/2
  Product14/1 -> Fy2/1
  Trigonometric Function15/1 -> Product14/1
  Product16/1 -> Product15/2, Product14/2
  Product15/1 -> Fx2/1
  alpha2/1 -> Trigonometric Function13/1, Trigonometric Function15/1
  Trigonometric Function13/1 -> Product15/1
  [ptoForce4] -> Product11/1

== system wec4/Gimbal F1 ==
  Assignment : Assignment  DiagnosticForDimensions=Warning  IndexOptions=Index vector (dialog)  Indices=[4 5 6]  OutputSizes=1
  Assignment1 : Assignment  DiagnosticForDimensions=Warning  IndexOptions=Index vector (dialog)  Indices=[4 5 6]  OutputSizes=1
  Assignment2 : Assignment  DiagnosticForDimensions=Warning  IndexOptions=Index vector (dialog)  Indices=[4 5 6]  OutputSizes=1
  Assignment3 : Assignment  DiagnosticForDimensions=Warning  IndexOptions=Index vector (dialog)  Indices=2  OutputSizes=1
  Assignment4 : Assignment  DiagnosticForDimensions=Warning  IndexOptions=Index vector (dialog)  Indices=2  OutputSizes=1
  CONSTRAINT (Gimbal Joint) : sm_lib/Joints/Gimbal Joint  SenseConstraintForce=on  SenseConstraintForceX=off  SenseConstraintForceY=off  SenseConstraintForceZ=off  SenseConstraintTorque=on  SenseConstraintTorqueX=off  SenseConstraintTorqueY=off  SenseConstraintTorqueZ=off  SenseTotalForce=off  SenseTotalForceX=off  SenseTotalForceY=off  SenseTotalForceZ=off  SenseTotalTorque=off  SenseTotalTorqueX=off  SenseTotalTorqueY=off  SenseTotalTorqueZ=off  CompositeWrenchDir=BaseOnFollower  CompositeWrenchFrame=BaseFrame  RxEquilibriumPosition=0  RxEquilibriumPositionUnits=rad  RxSpringStiffness=top_const_k  RxSpringStiffnessUnits=N*m/rad  RxDampingCoefficient=top_const_c  RxDampingCoefficientUnits=N*m/(rad/s)  RxTorqueActuationMode=NoTorque  RxMotionActuationMode=ComputedMotion  RxSensePosition=on  RxSenseVelocity=on  RxSenseAcceleration=on  RxSenseTorqueForce=off  RxPositionTargetSpecify=off  RxPositionTargetPriority=High  RxPositionTargetValue=0  RxPositionTargetValueUnits=deg  RxVelocityTargetSpecify=off  RxVelocityTargetPriority=High  RxVelocityTargetValue=0  RxVelocityTargetValueUnits=deg/s  RyEquilibriumPosition=0  RyEquilibriumPositionUnits=rad  RySpringStiffness=top_const_k  RySpringStiffnessUnits=N*m/rad  RyDampingCoefficient=top_const_c  RyDampingCoefficientUnits=N*m/(rad/s)  RyTorqueActuationMode=NoTorque  RyMotionActuationMode=ComputedMotion  RySensePosition=on  RySenseVelocity=on  RySenseAcceleration=on  RySenseTorqueForce=off  RyPositionTargetSpecify=off  RyPositionTargetPriority=High  RyPositionTargetValue=0  RyPositionTargetValueUnits=deg  RyVelocityTargetSpecify=off  RyVelocityTargetPriority=High  RyVelocityTargetValue=0  RyVelocityTargetValueUnits=deg/s  RzEquilibriumPosition=0  RzEquilibriumPositionUnits=rad  RzSpringStiffness=top_const_k  RzSpringStiffnessUnits=N*m/rad  RzDampingCoefficient=top_const_c  RzDampingCoefficientUnits=N*m/(rad/s)  RzTorqueActuationMode=NoTorque  RzMotionActuationMode=ComputedMotion  RzSensePosition=on  RzSenseVelocity=on  RzSenseAcceleration=on  RzSenseTorqueForce=off  RzPositionTargetSpecify=off  RzPositionTargetPriority=High  RzPositionTargetValue=0  RzPositionTargetValueUnits=deg  RzVelocityTargetSpecify=off  RzVelocityTargetPriority=High  RzVelocityTargetValue=0  RzVelocityTargetValueUnits=deg/s
  Constant : Constant  Value=[0 0 0 0 0 0]
  Constant1 : Constant  Value=[0 0 0 0 0 0]
  Constant2 : Constant  Value=[0 0 0 0 0 0]
  Gain{1..5} (5 alike) : Gain  Gain=-1
  Mux : Mux  Inputs=2
  Mux1 : Mux
  Mux2 : Mux  Inputs=3
  Mux3 : Mux  Inputs=3
  Mux4 : Mux  Inputs=3
  PS-Simulink Converter{1..11} (11 alike) : nesl_utility/PS-Simulink Converter  PhysicalDomain=network_engine_domain  SubClassName=ps_output  LeftPortType=input  RightPortType=output  PseudoPeriodic=off  Frequencies=[]  Unit=1  AffineConversion=off
  Rigid Transform (Position) : sm_lib/Frames and Transforms/Rigid Transform  TranslationMethod=Cartesian  TranslationStandardOffset=0  TranslationLengthUnit=m  TranslationStandardAxis=+Z  TranslationCartesianOffset=constraint.initDisp.initLinDisp+constraint.loc  TranslationROffset=0  TranslationROffsetUnits=m  TranslationZOffset=0  TranslationZOffsetUnits=m  TranslationThetaOffset=0  TranslationThetaOffsetUnits=deg  RotationMethod=None  RotationAngleUnits=rad  RotationStandardAxis=+Y  RotationAngle=0  RotationArbitraryAxis=[0 1 0]  FollAlignAxisA=+X  BaseAlignAxisA=+Y  FollAlignAxisB=+Y  BaseAlignAxisB=+Z  RotationSequenceAxes=FollowerAxes  RotationSequence=XYX  RotationSequenceAngles=[0 0 0]  RotationSequenceAnglesUnits=deg  RotationMatrix=[1 0 0; 0 1 0; 0 0 1]
  Rigid Transform (Position)1 : sm_lib/Frames and Transforms/Rigid Transform  TranslationMethod=Cartesian  TranslationStandardOffset=0  TranslationLengthUnit=m  TranslationStandardAxis=+Z  TranslationCartesianOffset=constraint.initDisp.initLinDisp+constraint.loc  TranslationROffset=0  TranslationROffsetUnits=m  TranslationZOffset=0  TranslationZOffsetUnits=m  TranslationThetaOffset=0  TranslationThetaOffsetUnits=deg  RotationMethod=None  RotationAngleUnits=rad  RotationStandardAxis=+Y  RotationAngle=0  RotationArbitraryAxis=[0 1 0]  FollAlignAxisA=+X  BaseAlignAxisA=+Y  FollAlignAxisB=+Y  BaseAlignAxisB=+Z  RotationSequenceAxes=FollowerAxes  RotationSequence=XYX  RotationSequenceAngles=[0 0 0]  RotationSequenceAnglesUnits=deg  RotationMatrix=[1 0 0; 0 1 0; 0 0 1]
  Rigid Transform (90 X) : sm_lib/Frames and Transforms/Rigid Transform  TranslationMethod=None  TranslationStandardOffset=0  TranslationLengthUnit=m  TranslationStandardAxis=+Z  TranslationCartesianOffset=constraint.loc  TranslationROffset=0  TranslationROffsetUnits=m  TranslationZOffset=0  TranslationZOffsetUnits=m  TranslationThetaOffset=0  TranslationThetaOffsetUnits=deg  RotationMethod=StandardAxis  RotationAngleUnits=deg  RotationStandardAxis=+X  RotationAngle=90  RotationArbitraryAxis=[0 1 0]  FollAlignAxisA=+X  BaseAlignAxisA=+Y  FollAlignAxisB=+Y  BaseAlignAxisB=+Z  RotationSequenceAxes=FollowerAxes  RotationSequence=XYX  RotationSequenceAngles=[0 0 0]  RotationSequenceAnglesUnits=deg  RotationMatrix=[1 0 0; 0 1 0; 0 0 1]
  Rigid Transform (90 X)1 : sm_lib/Frames and Transforms/Rigid Transform  TranslationMethod=None  TranslationStandardOffset=0  TranslationLengthUnit=m  TranslationStandardAxis=+Z  TranslationCartesianOffset=constraint.loc  TranslationROffset=0  TranslationROffsetUnits=m  TranslationZOffset=0  TranslationZOffsetUnits=m  TranslationThetaOffset=0  TranslationThetaOffsetUnits=deg  RotationMethod=StandardAxis  RotationAngleUnits=deg  RotationStandardAxis=+X  RotationAngle=90  RotationArbitraryAxis=[0 1 0]  FollAlignAxisA=+X  BaseAlignAxisA=+Y  FollAlignAxisB=+Y  BaseAlignAxisB=+Z  RotationSequenceAxes=FollowerAxes  RotationSequence=XYX  RotationSequenceAngles=[0 0 0]  RotationSequenceAnglesUnits=deg  RotationMatrix=[1 0 0; 0 1 0; 0 0 1]
  Rigid Transform (Orientation) : sm_lib/Frames and Transforms/Rigid Transform  TranslationMethod=None  TranslationStandardOffset=0  TranslationLengthUnit=m  TranslationStandardAxis=+Z  TranslationCartesianOffset=constraint.loc  TranslationROffset=0  TranslationROffsetUnits=m  TranslationZOffset=0  TranslationZOffsetUnits=m  TranslationThetaOffset=0  TranslationThetaOffsetUnits=deg  RotationMethod=RotationMatrix  RotationAngleUnits=rad  RotationStandardAxis=+Y  RotationAngle=0  RotationArbitraryAxis=[0 1 0]  FollAlignAxisA=+X  BaseAlignAxisA=+Y  FollAlignAxisB=+Y  BaseAlignAxisB=+Z  RotationSequenceAxes=FollowerAxes  RotationSequence=XYX  RotationSequenceAngles=[0 0 0]  RotationSequenceAnglesUnits=deg  RotationMatrix=constraint.orientation.rotationMatrix
  Rigid Transform (Orientation)1 : sm_lib/Frames and Transforms/Rigid Transform  TranslationMethod=None  TranslationStandardOffset=0  TranslationLengthUnit=m  TranslationStandardAxis=+Z  TranslationCartesianOffset=constraint.loc  TranslationROffset=0  TranslationROffsetUnits=m  TranslationZOffset=0  TranslationZOffsetUnits=m  TranslationThetaOffset=0  TranslationThetaOffsetUnits=deg  RotationMethod=RotationMatrix  RotationAngleUnits=rad  RotationStandardAxis=+Y  RotationAngle=0  RotationArbitraryAxis=[0 1 0]  FollAlignAxisA=+X  BaseAlignAxisA=+Y  FollAlignAxisB=+Y  BaseAlignAxisB=+Z  RotationSequenceAxes=FollowerAxes  RotationSequence=XYX  RotationSequenceAngles=[0 0 0]  RotationSequenceAnglesUnits=deg  RotationMatrix=constraint.orientation.rotationMatrix
  Selector : Selector  InputPortWidth=3  IndexOptions=Index vector (dialog)  Indices=[1 3 2]  OutputSizes=1
  Selector1 : Selector  InputPortWidth=3  IndexOptions=Index vector (dialog)  Indices=[2]  OutputSizes=1
  Selector2 : Selector  InputPortWidth=3  IndexOptions=Index vector (dialog)  Indices=[1 3 2]  OutputSizes=1
  Selector3 : Selector  InputPortWidth=3  IndexOptions=Index vector (dialog)  Indices=[2]  OutputSizes=1
  output : ToWorkspace  VariableName=constraint5_out  SaveFormat=Structure With Time  SampleTime=-1
  F : PMIOPort  Port=1  Side=Right
  B : PMIOPort  Port=2  Side=Left
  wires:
  Assignment4/1 -> Mux/2
  PS-Simulink Converter4/1 -> Selector2/1
  Gain4/1 -> Assignment4/2
  Selector3/1 -> Gain4/1
  Selector2/1 -> Assignment4/1, Selector3/1
  Assignment3/1 -> Mux/1
  Gain3/1 -> Assignment3/2
  Selector1/1 -> Gain3/1
  Selector/1 -> Selector1/1, Assignment3/1
  PS-Simulink Converter3/1 -> Selector/1
  Mux3/1 -> Assignment1/2
  Mux4/1 -> Assignment/2
  Constant/1 -> Assignment/1
  Constant1/1 -> Assignment1/1
  Constant2/1 -> Assignment2/1
  Assignment2/1 -> Mux1/3  "acceleration"
  Assignment1/1 -> Mux1/2  "velocity"
  Assignment/1 -> Mux1/1  "position"
  Mux/1 -> Mux1/4  "Constraint Forces"
  Mux1/1 -> output/1
  PS-Simulink Converter5/1 -> Gain5/1
  Gain5/1 -> Mux2/2
  PS-Simulink Converter6/1 -> Mux2/3
  PS-Simulink Converter7/1 -> Mux2/1
  Mux2/1 -> Assignment2/2
  PS-Simulink Converter2/1 -> Gain2/1
  Gain2/1 -> Mux3/2
  PS-Simulink Converter8/1 -> Mux3/3
  PS-Simulink Converter9/1 -> Mux3/1
  PS-Simulink Converter11/1 -> Gain1/1
  Gain1/1 -> Mux4/2
  PS-Simulink Converter1/1 -> Mux4/1
  PS-Simulink Converter10/1 -> Mux4/3
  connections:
  Rigid Transform (Position)1/LConn1 -- F/RConn1
  Rigid Transform (Position)1/RConn1 -- Rigid Transform (Orientation)1/LConn1
  Rigid Transform (Orientation)1/RConn1 -- Rigid Transform (90 X)1/LConn1
  Rigid Transform (Orientation)/RConn1 -- Rigid Transform (90 X)/LConn1
  Rigid Transform (Position)/RConn1 -- Rigid Transform (Orientation)/LConn1
  Rigid Transform (Position)/LConn1 -- B/RConn1
  PS-Simulink Converter4/LConn1 -- CONSTRAINT (Gimbal Joint)/RConn12
  PS-Simulink Converter3/LConn1 -- CONSTRAINT (Gimbal Joint)/RConn11
  PS-Simulink Converter5/LConn1 -- CONSTRAINT (Gimbal Joint)/RConn10
  PS-Simulink Converter6/LConn1 -- CONSTRAINT (Gimbal Joint)/RConn7
  PS-Simulink Converter7/LConn1 -- CONSTRAINT (Gimbal Joint)/RConn4
  CONSTRAINT (Gimbal Joint)/LConn1 -- Rigid Transform (90 X)/RConn1
  PS-Simulink Converter2/LConn1 -- CONSTRAINT (Gimbal Joint)/RConn9
  CONSTRAINT (Gimbal Joint)/RConn6 -- PS-Simulink Converter8/LConn1
  PS-Simulink Converter9/LConn1 -- CONSTRAINT (Gimbal Joint)/RConn3
  CONSTRAINT (Gimbal Joint)/RConn2 -- PS-Simulink Converter1/LConn1
  CONSTRAINT (Gimbal Joint)/RConn5 -- PS-Simulink Converter10/LConn1
  PS-Simulink Converter11/LConn1 -- CONSTRAINT (Gimbal Joint)/RConn8
  Rigid Transform (90 X)1/RConn1 -- CONSTRAINT (Gimbal Joint)/RConn1
